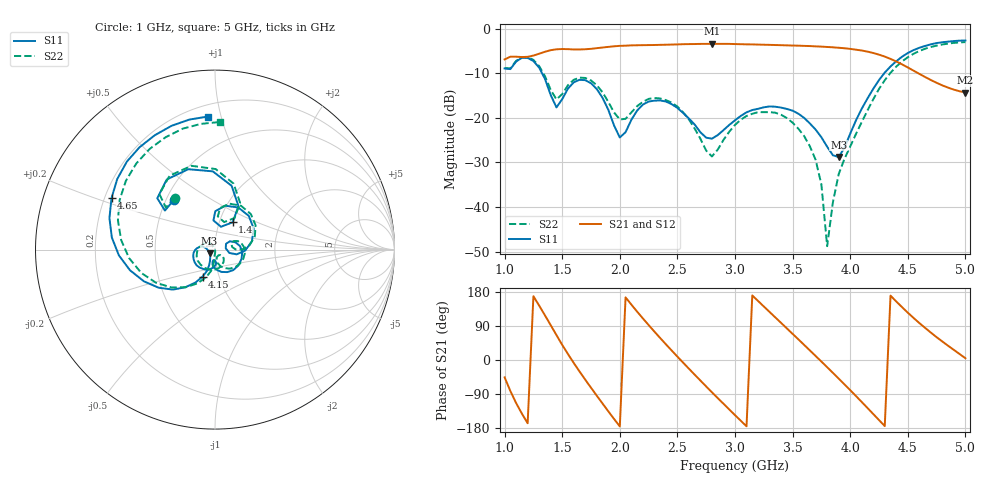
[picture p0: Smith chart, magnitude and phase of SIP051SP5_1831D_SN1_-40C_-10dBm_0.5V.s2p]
# GHz  S  dB  R  50
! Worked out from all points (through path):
!   81 points, 1 GHz to 5 GHz, reference 50 ohm
!   highest |S21| = -3.34 dB at 2.8 GHz (marker M1); lowest = -14.3 dB at 5 GHz (marker M2)
!   lowest |S11| = -28.8 dB at 3.9 GHz (marker M3), VSWR 1.08, Z = 47 - j1.91 ohm
!   |S11| at or under -10 dB: 1.326 GHz to 4.294 GHz (2.968 GHz wide, 106 % of centre)
!   |S22| runs from -48.8 to -3.0 dB; largest |S21 - S12| = 0.0019
!   S11 on the Smith chart (normalised r, x): 1 GHz: 0.55, +0.35; 1.4 GHz: 1.16, +0.36; 4.15 GHz: 0.83, -0.26; 4.65 GHz: 0.23, +0.22; 5 GHz: 0.27, +0.91
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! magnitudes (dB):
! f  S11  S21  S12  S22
! 1 GHz  -8.9  -6.8  -6.8  -8.8
! 1.25 GHz  -7.2  -6.0  -6.0  -7.0
! 1.4 GHz  -14.8  -4.8  -4.8  -13.7
! 1.45 GHz  -17.6  -4.6  -4.6  -15.8
! 1.7 GHz  -11.5  -4.6  -4.6  -11.0
! 1.85 GHz  -15.5  -4.2  -4.2  -14.2
! 2 GHz  -24.4  -3.8  -3.8  -20.3
! 2.2 GHz  -17.0  -3.6  -3.6  -16.4
! 2.35 GHz  -16.1  -3.6  -3.6  -15.6
! 2.55 GHz  -18.9  -3.4  -3.4  -18.7
! 2.8 GHz  -24.6  -3.3  -3.3  -28.6
! 3 GHz  -20.5  -3.4  -3.4  -21.6
! 3.4 GHz  -17.7  -3.6  -3.6  -19.3
! 3.6 GHz  -20.0  -3.8  -3.8  -24.1
! 3.7 GHz  -22.6  -3.9  -3.9  -29.4
! 3.75 GHz  -24.3  -4.0  -4.0  -35.0
! 3.8 GHz  -26.5  -4.0  -4.0  -48.8
! 3.9 GHz  -28.8  -4.2  -4.2  -32.6
! 4.15 GHz  -15.6  -5.1  -5.1  -18.3
! 4.35 GHz  -8.4  -6.7  -6.7  -9.9
! 4.65 GHz  -3.8  -10.8  -10.8  -4.5
! 5 GHz  -2.6  -14.3  -14.3  -3.0
